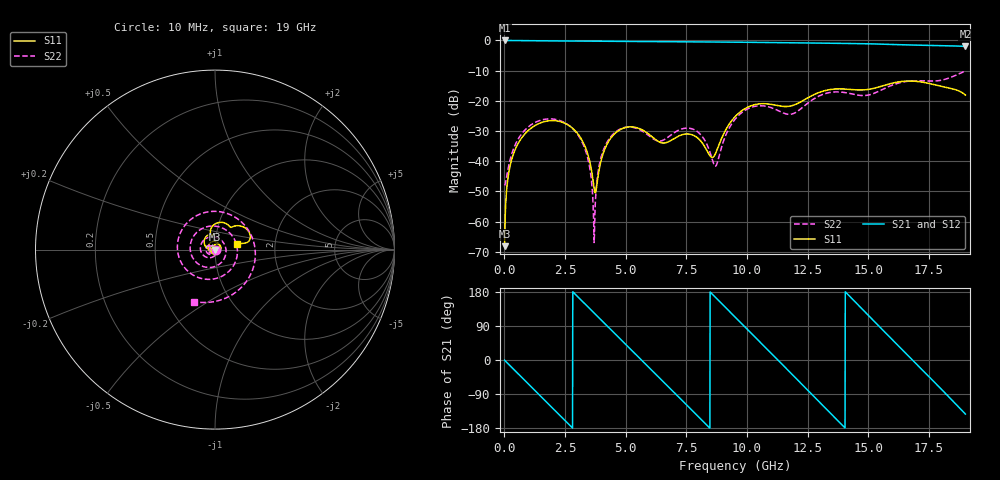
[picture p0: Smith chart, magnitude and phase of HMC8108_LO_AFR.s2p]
! Analog Devices, Inc.
! 1 Analog Way
! Wilmington, MA 01887
! http://www.analog.com
! Date:  2021-09-07 NN
! Board Name:  EV1HMC8108LC5 Revision A with HMC8108LC5 installed
! File Description:  Automatic Fixture Removal S-Parameters for LO Port connector and board loss de-embedding
! File Generation:  Calibrated Network Analyzer
! Chip Part Number:  HMC8108
! Chip Description:  X-Band, GaAs, MMIC, Low Noise Converter
! Chip Frequency:  9 to 10 GHz
! Chip Package:  LCC, 5 x 5 x 1.12 mm
! LO Port:  HMC8108LC5 removed and end of trace left open
! Note:
!  Analog Devices supplies this data as a sample of measured data at the evaluation board
!  ports for this product.  Your particular data for this product may vary.
!  Analog Devices reserves the right to change this data at anytime.
!  All lines below in this file are as is from the Network Analyzer.
!Agilent Technologies,N5245A,MY52451809,A.10.47.06
!Automatic Fixture Removal (AFR)
!Date: Friday, August 27, 2021 11:17:57 PM
!S2P File: Measurements: S11,S21,S12,S22:
# MHz S  RI  R 50
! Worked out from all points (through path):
!   1900 points, 10 MHz to 19 GHz, reference 50 ohm
!   highest |S21| = 0.00 dB at 10 MHz (marker M1); lowest = -2.0 dB at 19 GHz (marker M2)
!   group delay of S21, straight-line fit = 179 ps
!   lowest |S11| = -68.1 dB at 10 MHz (marker M3), VSWR 1.00, Z = 50 - j0.036 ohm
!   |S11| at or under -10 dB: start of sweep to end of sweep
!   |S22| runs from -66.9 to -10.1 dB; largest |S21 - S12| = 1.4e-15
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10  0.000159 -0.00036  1 -0.0112  1 -0.0112  0.00394 -0.000454
250  -0.00316 -0.0083  0.9591 -0.2758  0.9591 -0.2758  0.00162 -0.011
840  -0.0267 -0.00919  0.5853 -0.8017  0.5853 -0.8017  -0.0186 -0.0269
1830  -0.0233 0.0406  -0.4483 -0.8765  -0.4483 -0.8765  -0.0502 -0.00289
3180  0.0211 0.0093  -0.8985 0.3798  -0.8985 0.3798  -0.00876 0.0199
3700  0.00284 0.00214  -0.544 0.8055  -0.544 0.8055  -0.000443 8.98e-05
3980  -0.00527 0.00853  -0.2712 0.9313  -0.2712 0.9313  -0.00438 -0.0106
4470  -0.00362 0.0264  0.2487 0.9339  0.2487 0.9339  -0.0204 -0.019
5450  0.0323 0.0159  0.9362 0.2124  0.9362 0.2124  -0.035 0.00169
6340  0.00674 -0.0203  0.6883 -0.6619  0.6883 -0.6619  -0.0216 0.00168
7230  -0.0259 0.0063  -0.1751 -0.9332  -0.1751 -0.9332  -0.0334 0.000676
8180  -0.00659 0.0183  -0.8951 -0.3027  -0.8951 -0.3027  -0.0132 0.0212
8710  -0.0131 0.004  -0.9092 0.2487  -0.9092 0.2487  0.00815 0.00171
9510  -0.0523 0.0167  -0.3706 0.8609  -0.3706 0.8609  -0.0223 -0.0445
11170  -0.0169 0.0834  0.9187 0.1069  0.9187 0.1069  -0.0135 0.0712
12670  -0.0208 0.1201  -0.00937 -0.91  -0.00937 -0.91  -0.0252 -0.0993
14150  0.0726 0.1378  -0.8855 0.1015  -0.8855 0.1015  -0.0404 0.1286
15060  0.0931 0.1254  -0.3581 0.8039  -0.3581 0.8039  0.1246 -0.0217
15840  0.1356 0.1326  0.3892 0.7688  0.3892 0.7688  -0.0487 -0.1653
17120  0.1966 0.0657  0.7893 -0.2752  0.7893 -0.2752  -0.106 0.1871
18080  0.1681 0.0368  0.1197 -0.8142  0.1197 -0.8142  0.2231 0.00527
19000  0.1215 0.0289  -0.6337 -0.4835  -0.6337 -0.4835  -0.1161 -0.2898
